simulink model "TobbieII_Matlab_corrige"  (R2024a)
settings: Solver=VariableStepAuto  StartTime=0.0  StopTime=10  RelTol=1e-3
model workspace: external: MATLAB File (data not in the file)
undefined symbols (not defined in the file or in its folder): deg, kg, m, mm, N, s, smiData, X, Y, Z
libraries: sm_lib x63, fl_lib x16, nesl_utility x9, ee_lib x2, simulink x1
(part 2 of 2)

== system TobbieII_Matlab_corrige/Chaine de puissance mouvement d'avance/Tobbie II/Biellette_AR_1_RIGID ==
  ReferenceFrame : sm_lib/Frames and Transforms/Reference Frame
  Solid : sm_lib/Body Elements/File Solid  ExtGeomFileName=Biellette AR_Défaut_sldprt.STEP  UnitType=FromFile  ExtGeomFileUnits=m  StepReaderType=HEX  ExportConvexHullGeometry=off  InertiaType=Custom  BasedOnType=DensityFromFile  Density=1000  DensityUnits=kg/m^3  Mass=smiData.Solid(2).mass  MassUnits=kg  CenterOfMass=smiData.Solid(2).CoM  CenterOfMassUnits=mm  MomentsOfInertia=smiData.Solid(2).MoI  MomentsOfInertiaUnits=kg*mm^2  ProductsOfInertia=smiData.Solid(2).PoI  ProductsOfInertiaUnits=kg*mm^2  GraphicType=FromGeometry  MarkerShape=Sphere  MarkerSize=10  GraphicVisPropType=SimpleVisualProperties  GraphicDiffuseColor=smiData.Solid(2).color  GraphicOpacity=smiData.Solid(2).opacity  GraphicSpecularColor=[0.5 0.5 0.5 1.0]  GraphicAmbientColor=[0.15 0.15 0.15 1.0]  GraphicEmissiveColor=[0.0 0.0 0.0 1.0]  GraphicShininess=75  DoExposeReferenceFrame=on  SerializedFrames=<Frames/>
  Transform : sm_lib/Frames and Transforms/Rigid Transform  RotationMethod=ArbitraryAxis  FollAlignAxisA=+X  BaseAlignAxisA=+Y  FollAlignAxisB=+Y  BaseAlignAxisB=+Z  RotationStandardAxis=+Z  RotationAngle=smiData.RigidTransform(23).angle  RotationAngleUnits=rad  RotationArbitraryAxis=smiData.RigidTransform(23).axis  RotationSequenceAxes=FollowerAxes  RotationSequence=XYX  RotationSequenceAngles=[0 0 0]  RotationSequenceAnglesUnits=deg  RotationMatrix=[1 0 0;0 1 0;0 0 1]  Quaternion=[1 0 0 0]  TranslationMethod=Cartesian  TranslationCartesianOffset=smiData.RigidTransform(23).translation  TranslationCartesianOffsetUnits=mm  TranslationStandardAxis=+Z  TranslationStandardOffset=0  TranslationStandardOffsetUnits=m  TranslationROffset=0  TranslationROffsetUnits=m  TranslationThetaOffset=0  TranslationThetaOffsetUnits=deg  TranslationZOffset=0  TranslationZOffsetUnits=m
  Transform1 : sm_lib/Frames and Transforms/Rigid Transform  RotationMethod=ArbitraryAxis  FollAlignAxisA=+X  BaseAlignAxisA=+Y  FollAlignAxisB=+Y  BaseAlignAxisB=+Z  RotationStandardAxis=+Z  RotationAngle=smiData.RigidTransform(26).angle  RotationAngleUnits=rad  RotationArbitraryAxis=smiData.RigidTransform(26).axis  RotationSequenceAxes=FollowerAxes  RotationSequence=XYX  RotationSequenceAngles=[0 0 0]  RotationSequenceAnglesUnits=deg  RotationMatrix=[1 0 0;0 1 0;0 0 1]  Quaternion=[1 0 0 0]  TranslationMethod=Cartesian  TranslationCartesianOffset=smiData.RigidTransform(26).translation  TranslationCartesianOffsetUnits=mm  TranslationStandardAxis=+Z  TranslationStandardOffset=0  TranslationStandardOffsetUnits=m  TranslationROffset=0  TranslationROffsetUnits=m  TranslationThetaOffset=0  TranslationThetaOffsetUnits=deg  TranslationZOffset=0  TranslationZOffsetUnits=m
  F1 : PMIOPort  Side=Left
  F : PMIOPort  Port=2  Side=Right
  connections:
  Solid/RConn1 -- ReferenceFrame/RConn1 -- Transform/LConn1 -- Transform1/LConn1
  Transform/RConn1 -- F/RConn1
  Transform1/RConn1 -- F1/RConn1

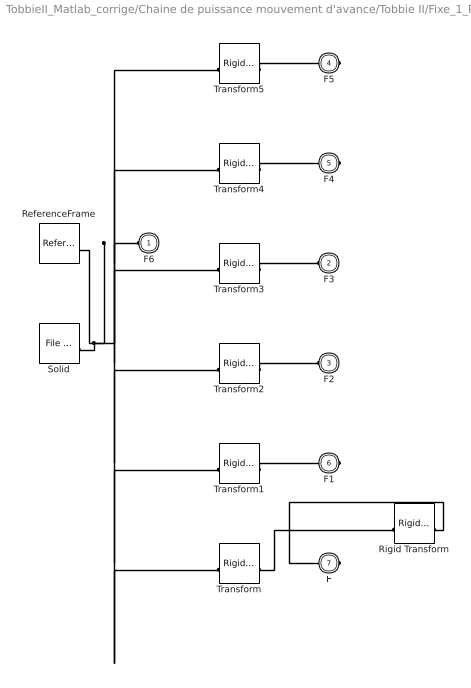
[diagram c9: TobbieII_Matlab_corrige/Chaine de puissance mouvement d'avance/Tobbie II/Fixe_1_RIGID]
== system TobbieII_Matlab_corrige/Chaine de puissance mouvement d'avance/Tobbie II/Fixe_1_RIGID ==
  ReferenceFrame : sm_lib/Frames and Transforms/Reference Frame
  Rigid Transform : sm_lib/Frames and Transforms/Rigid Transform  RotationMethod=RotationSequence  FollAlignAxisA=+X  BaseAlignAxisA=+Y  FollAlignAxisB=+Y  BaseAlignAxisB=+Z  RotationStandardAxis=+Z  RotationAngle=0  RotationAngleUnits=deg  RotationArbitraryAxis=[0 0 1]  RotationSequenceAxes=FollowerAxes  RotationSequence=XYZ  RotationSequenceAngles=[90 0 90]  RotationSequenceAnglesUnits=deg  RotationMatrix=[1 0 0;0 1 0;0 0 1]  Quaternion=[1 0 0 0]  TranslationMethod=Cartesian  TranslationCartesianOffset=[-2 0 0]  TranslationCartesianOffsetUnits=mm  TranslationStandardAxis=+Z  TranslationStandardOffset=0  TranslationStandardOffsetUnits=m  TranslationROffset=0  TranslationROffsetUnits=m  TranslationThetaOffset=0  TranslationThetaOffsetUnits=deg  TranslationZOffset=0  TranslationZOffsetUnits=m
  Solid : sm_lib/Body Elements/File Solid  ExtGeomFileName=Fixe_Défaut_sldprt.STEP  UnitType=FromFile  ExtGeomFileUnits=m  StepReaderType=HEX  ExportConvexHullGeometry=off  InertiaType=Custom  BasedOnType=DensityFromFile  Density=1000  DensityUnits=kg/m^3  Mass=smiData.Solid(5).mass  MassUnits=kg  CenterOfMass=smiData.Solid(5).CoM  CenterOfMassUnits=mm  MomentsOfInertia=smiData.Solid(5).MoI  MomentsOfInertiaUnits=kg*mm^2  ProductsOfInertia=smiData.Solid(5).PoI  ProductsOfInertiaUnits=kg*mm^2  GraphicType=FromGeometry  MarkerShape=Sphere  MarkerSize=10  GraphicVisPropType=SimpleVisualProperties  GraphicDiffuseColor=smiData.Solid(5).color  GraphicOpacity=smiData.Solid(5).opacity  GraphicSpecularColor=[0.5 0.5 0.5 1.0]  GraphicAmbientColor=[0.15 0.15 0.15 1.0]  GraphicEmissiveColor=[0.0 0.0 0.0 1.0]  GraphicShininess=75  DoExposeReferenceFrame=on  SerializedFrames=<Frames/>
  Transform : sm_lib/Frames and Transforms/Rigid Transform  RotationMethod=ArbitraryAxis  FollAlignAxisA=+X  BaseAlignAxisA=+Y  FollAlignAxisB=+Y  BaseAlignAxisB=+Z  RotationStandardAxis=+Z  RotationAngle=smiData.RigidTransform(3).angle  RotationAngleUnits=rad  RotationArbitraryAxis=smiData.RigidTransform(3).axis  RotationSequenceAxes=FollowerAxes  RotationSequence=XYX  RotationSequenceAngles=[0 0 0]  RotationSequenceAnglesUnits=deg  RotationMatrix=[1 0 0;0 1 0;0 0 1]  Quaternion=[1 0 0 0]  TranslationMethod=Cartesian  TranslationCartesianOffset=smiData.RigidTransform(3).translation  TranslationCartesianOffsetUnits=mm  TranslationStandardAxis=+Z  TranslationStandardOffset=0  TranslationStandardOffsetUnits=m  TranslationROffset=0  TranslationROffsetUnits=m  TranslationThetaOffset=0  TranslationThetaOffsetUnits=deg  TranslationZOffset=0  TranslationZOffsetUnits=m
  Transform1 : sm_lib/Frames and Transforms/Rigid Transform  RotationMethod=ArbitraryAxis  FollAlignAxisA=+X  BaseAlignAxisA=+Y  FollAlignAxisB=+Y  BaseAlignAxisB=+Z  RotationStandardAxis=+Z  RotationAngle=smiData.RigidTransform(9).angle  RotationAngleUnits=rad  RotationArbitraryAxis=smiData.RigidTransform(9).axis  RotationSequenceAxes=FollowerAxes  RotationSequence=XYX  RotationSequenceAngles=[0 0 0]  RotationSequenceAnglesUnits=deg  RotationMatrix=[1 0 0;0 1 0;0 0 1]  Quaternion=[1 0 0 0]  TranslationMethod=Cartesian  TranslationCartesianOffset=smiData.RigidTransform(9).translation  TranslationCartesianOffsetUnits=mm  TranslationStandardAxis=+Z  TranslationStandardOffset=0  TranslationStandardOffsetUnits=m  TranslationROffset=0  TranslationROffsetUnits=m  TranslationThetaOffset=0  TranslationThetaOffsetUnits=deg  TranslationZOffset=0  TranslationZOffsetUnits=m
  Transform2 : sm_lib/Frames and Transforms/Rigid Transform  RotationMethod=ArbitraryAxis  FollAlignAxisA=+X  BaseAlignAxisA=+Y  FollAlignAxisB=+Y  BaseAlignAxisB=+Z  RotationStandardAxis=+Z  RotationAngle=smiData.RigidTransform(18).angle  RotationAngleUnits=rad  RotationArbitraryAxis=smiData.RigidTransform(18).axis  RotationSequenceAxes=FollowerAxes  RotationSequence=XYX  RotationSequenceAngles=[0 0 0]  RotationSequenceAnglesUnits=deg  RotationMatrix=[1 0 0;0 1 0;0 0 1]  Quaternion=[1 0 0 0]  TranslationMethod=Cartesian  TranslationCartesianOffset=smiData.RigidTransform(18).translation  TranslationCartesianOffsetUnits=mm  TranslationStandardAxis=+Z  TranslationStandardOffset=0  TranslationStandardOffsetUnits=m  TranslationROffset=0  TranslationROffsetUnits=m  TranslationThetaOffset=0  TranslationThetaOffsetUnits=deg  TranslationZOffset=0  TranslationZOffsetUnits=m
  Transform3 : sm_lib/Frames and Transforms/Rigid Transform  RotationMethod=ArbitraryAxis  FollAlignAxisA=+X  BaseAlignAxisA=+Y  FollAlignAxisB=+Y  BaseAlignAxisB=+Z  RotationStandardAxis=+Z  RotationAngle=smiData.RigidTransform(20).angle  RotationAngleUnits=rad  RotationArbitraryAxis=smiData.RigidTransform(20).axis  RotationSequenceAxes=FollowerAxes  RotationSequence=XYX  RotationSequenceAngles=[0 0 0]  RotationSequenceAnglesUnits=deg  RotationMatrix=[1 0 0;0 1 0;0 0 1]  Quaternion=[1 0 0 0]  TranslationMethod=Cartesian  TranslationCartesianOffset=smiData.RigidTransform(20).translation  TranslationCartesianOffsetUnits=mm  TranslationStandardAxis=+Z  TranslationStandardOffset=0  TranslationStandardOffsetUnits=m  TranslationROffset=0  TranslationROffsetUnits=m  TranslationThetaOffset=0  TranslationThetaOffsetUnits=deg  TranslationZOffset=0  TranslationZOffsetUnits=m
  Transform4 : sm_lib/Frames and Transforms/Rigid Transform  RotationMethod=ArbitraryAxis  FollAlignAxisA=+X  BaseAlignAxisA=+Y  FollAlignAxisB=+Y  BaseAlignAxisB=+Z  RotationStandardAxis=+Z  RotationAngle=smiData.RigidTransform(21).angle  RotationAngleUnits=rad  RotationArbitraryAxis=smiData.RigidTransform(21).axis  RotationSequenceAxes=FollowerAxes  RotationSequence=XYX  RotationSequenceAngles=[0 0 0]  RotationSequenceAnglesUnits=deg  RotationMatrix=[1 0 0;0 1 0;0 0 1]  Quaternion=[1 0 0 0]  TranslationMethod=Cartesian  TranslationCartesianOffset=smiData.RigidTransform(21).translation  TranslationCartesianOffsetUnits=mm  TranslationStandardAxis=+Z  TranslationStandardOffset=0  TranslationStandardOffsetUnits=m  TranslationROffset=0  TranslationROffsetUnits=m  TranslationThetaOffset=0  TranslationThetaOffsetUnits=deg  TranslationZOffset=0  TranslationZOffsetUnits=m
  Transform5 : sm_lib/Frames and Transforms/Rigid Transform  RotationMethod=ArbitraryAxis  FollAlignAxisA=+X  BaseAlignAxisA=+Y  FollAlignAxisB=+Y  BaseAlignAxisB=+Z  RotationStandardAxis=+Z  RotationAngle=smiData.RigidTransform(25).angle  RotationAngleUnits=rad  RotationArbitraryAxis=smiData.RigidTransform(25).axis  RotationSequenceAxes=FollowerAxes  RotationSequence=XYX  RotationSequenceAngles=[0 0 0]  RotationSequenceAnglesUnits=deg  RotationMatrix=[1 0 0;0 1 0;0 0 1]  Quaternion=[1 0 0 0]  TranslationMethod=Cartesian  TranslationCartesianOffset=smiData.RigidTransform(25).translation  TranslationCartesianOffsetUnits=mm  TranslationStandardAxis=+Z  TranslationStandardOffset=0  TranslationStandardOffsetUnits=m  TranslationROffset=0  TranslationROffsetUnits=m  TranslationThetaOffset=0  TranslationThetaOffsetUnits=deg  TranslationZOffset=0  TranslationZOffsetUnits=m
  F6 : PMIOPort  Side=Left
  F3 : PMIOPort  Port=2  Side=Left
  F2 : PMIOPort  Port=3  Side=Left
  F5 : PMIOPort  Port=4  Side=Right
  F4 : PMIOPort  Port=5  Side=Right
  F1 : PMIOPort  Port=6  Side=Right
  F : PMIOPort  Port=7  Side=Right
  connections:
  Solid/RConn1 -- ReferenceFrame/RConn1 -- Transform/LConn1 -- Transform1/LConn1 -- Transform2/LConn1 -- Transform3/LConn1 -- Transform4/LConn1 -- Transform5/LConn1 -- F6/RConn1
  Transform/RConn1 -- Rigid Transform/LConn1
  Transform1/RConn1 -- F1/RConn1
  Transform2/RConn1 -- F2/RConn1
  Transform3/RConn1 -- F3/RConn1
  Transform4/RConn1 -- F4/RConn1
  Transform5/RConn1 -- F5/RConn1
  Rigid Transform/RConn1 -- F/RConn1

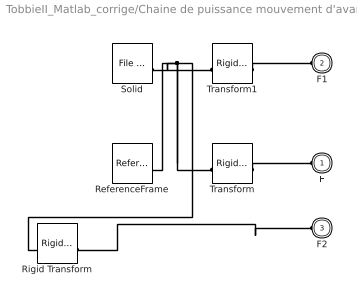
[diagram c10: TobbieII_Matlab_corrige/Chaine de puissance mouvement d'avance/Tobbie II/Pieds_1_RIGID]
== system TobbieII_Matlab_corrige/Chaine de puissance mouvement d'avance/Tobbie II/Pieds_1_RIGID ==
  ReferenceFrame : sm_lib/Frames and Transforms/Reference Frame
  Rigid Transform : sm_lib/Frames and Transforms/Rigid Transform  RotationMethod=None  FollAlignAxisA=+X  BaseAlignAxisA=+Y  FollAlignAxisB=+Y  BaseAlignAxisB=+Z  RotationStandardAxis=+Z  RotationAngle=0  RotationAngleUnits=deg  RotationArbitraryAxis=[0 0 1]  RotationSequenceAxes=FollowerAxes  RotationSequence=XYX  RotationSequenceAngles=[0 0 0]  RotationSequenceAnglesUnits=deg  RotationMatrix=[1 0 0;0 1 0;0 0 1]  Quaternion=[1 0 0 0]  TranslationMethod=Cartesian  TranslationCartesianOffset=[0 -42 0]  TranslationCartesianOffsetUnits=mm  TranslationStandardAxis=+Z  TranslationStandardOffset=0  TranslationStandardOffsetUnits=m  TranslationROffset=0  TranslationROffsetUnits=m  TranslationThetaOffset=0  TranslationThetaOffsetUnits=deg  TranslationZOffset=0  TranslationZOffsetUnits=m
  Solid : sm_lib/Body Elements/File Solid  ExtGeomFileName=Pieds_Défaut_sldprt.STEP  UnitType=FromFile  ExtGeomFileUnits=m  StepReaderType=HEX  ExportConvexHullGeometry=off  InertiaType=Custom  BasedOnType=DensityFromFile  Density=1000  DensityUnits=kg/m^3  Mass=smiData.Solid(7).mass  MassUnits=kg  CenterOfMass=smiData.Solid(7).CoM  CenterOfMassUnits=mm  MomentsOfInertia=smiData.Solid(7).MoI  MomentsOfInertiaUnits=kg*mm^2  ProductsOfInertia=smiData.Solid(7).PoI  ProductsOfInertiaUnits=kg*mm^2  GraphicType=FromGeometry  MarkerShape=Sphere  MarkerSize=10  GraphicVisPropType=SimpleVisualProperties  GraphicDiffuseColor=smiData.Solid(7).color  GraphicOpacity=smiData.Solid(7).opacity  GraphicSpecularColor=[0.5 0.5 0.5 1.0]  GraphicAmbientColor=[0.15 0.15 0.15 1.0]  GraphicEmissiveColor=[0.0 0.0 0.0 1.0]  GraphicShininess=75  DoExposeReferenceFrame=on  SerializedFrames=<Frames/>
  Transform : sm_lib/Frames and Transforms/Rigid Transform  RotationMethod=ArbitraryAxis  FollAlignAxisA=+X  BaseAlignAxisA=+Y  FollAlignAxisB=+Y  BaseAlignAxisB=+Z  RotationStandardAxis=+Z  RotationAngle=smiData.RigidTransform(2).angle  RotationAngleUnits=rad  RotationArbitraryAxis=smiData.RigidTransform(2).axis  RotationSequenceAxes=FollowerAxes  RotationSequence=XYX  RotationSequenceAngles=[0 0 0]  RotationSequenceAnglesUnits=deg  RotationMatrix=[1 0 0;0 1 0;0 0 1]  Quaternion=[1 0 0 0]  TranslationMethod=Cartesian  TranslationCartesianOffset=smiData.RigidTransform(2).translation  TranslationCartesianOffsetUnits=mm  TranslationStandardAxis=+Z  TranslationStandardOffset=0  TranslationStandardOffsetUnits=m  TranslationROffset=0  TranslationROffsetUnits=m  TranslationThetaOffset=0  TranslationThetaOffsetUnits=deg  TranslationZOffset=0  TranslationZOffsetUnits=m
  Transform1 : sm_lib/Frames and Transforms/Rigid Transform  RotationMethod=ArbitraryAxis  FollAlignAxisA=+X  BaseAlignAxisA=+Y  FollAlignAxisB=+Y  BaseAlignAxisB=+Z  RotationStandardAxis=+Z  RotationAngle=smiData.RigidTransform(8).angle  RotationAngleUnits=rad  RotationArbitraryAxis=smiData.RigidTransform(8).axis  RotationSequenceAxes=FollowerAxes  RotationSequence=XYX  RotationSequenceAngles=[0 0 0]  RotationSequenceAnglesUnits=deg  RotationMatrix=[1 0 0;0 1 0;0 0 1]  Quaternion=[1 0 0 0]  TranslationMethod=Cartesian  TranslationCartesianOffset=smiData.RigidTransform(8).translation  TranslationCartesianOffsetUnits=mm  TranslationStandardAxis=+Z  TranslationStandardOffset=0  TranslationStandardOffsetUnits=m  TranslationROffset=0  TranslationROffsetUnits=m  TranslationThetaOffset=0  TranslationThetaOffsetUnits=deg  TranslationZOffset=0  TranslationZOffsetUnits=m
  F : PMIOPort  Side=Left
  F1 : PMIOPort  Port=2  Side=Left
  F2 : PMIOPort  Port=3  Side=Left
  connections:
  Solid/RConn1 -- Rigid Transform/LConn1 -- Transform/LConn1 -- ReferenceFrame/RConn1 -- Transform1/LConn1
  Transform/RConn1 -- F/RConn1
  Transform1/RConn1 -- F1/RConn1
  Rigid Transform/RConn1 -- F2/RConn1

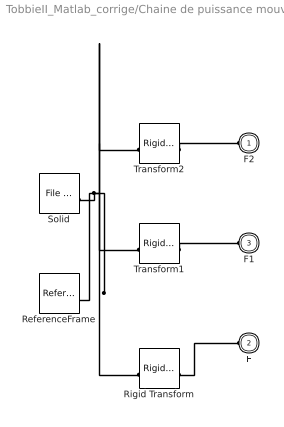
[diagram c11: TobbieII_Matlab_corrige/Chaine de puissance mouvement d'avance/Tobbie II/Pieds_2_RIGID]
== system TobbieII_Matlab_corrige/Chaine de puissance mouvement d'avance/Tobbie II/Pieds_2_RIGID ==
  ReferenceFrame : sm_lib/Frames and Transforms/Reference Frame
  Rigid Transform : sm_lib/Frames and Transforms/Rigid Transform  RotationMethod=StandardAxis  FollAlignAxisA=+X  BaseAlignAxisA=+Y  FollAlignAxisB=+Y  BaseAlignAxisB=+Z  RotationStandardAxis=+Z  RotationAngle=159.06  RotationAngleUnits=deg  RotationArbitraryAxis=[0 0 1]  RotationSequenceAxes=FollowerAxes  RotationSequence=XYX  RotationSequenceAngles=[0 0 0]  RotationSequenceAnglesUnits=deg  RotationMatrix=[1 0 0;0 1 0;0 0 1]  Quaternion=[1 0 0 0]  TranslationMethod=Cartesian  TranslationCartesianOffset=[0 -42 0]  TranslationCartesianOffsetUnits=mm  TranslationStandardAxis=+Z  TranslationStandardOffset=0  TranslationStandardOffsetUnits=m  TranslationROffset=0  TranslationROffsetUnits=m  TranslationThetaOffset=0  TranslationThetaOffsetUnits=deg  TranslationZOffset=0  TranslationZOffsetUnits=m
  Solid : sm_lib/Body Elements/File Solid  ExtGeomFileName=Pieds_Défaut_sldprt.STEP  UnitType=FromFile  ExtGeomFileUnits=m  StepReaderType=HEX  ExportConvexHullGeometry=off  InertiaType=Custom  BasedOnType=DensityFromFile  Density=1000  DensityUnits=kg/m^3  Mass=smiData.Solid(7).mass  MassUnits=kg  CenterOfMass=smiData.Solid(7).CoM  CenterOfMassUnits=mm  MomentsOfInertia=smiData.Solid(7).MoI  MomentsOfInertiaUnits=kg*mm^2  ProductsOfInertia=smiData.Solid(7).PoI  ProductsOfInertiaUnits=kg*mm^2  GraphicType=FromGeometry  MarkerShape=Sphere  MarkerSize=10  GraphicVisPropType=SimpleVisualProperties  GraphicDiffuseColor=smiData.Solid(7).color  GraphicOpacity=smiData.Solid(7).opacity  GraphicSpecularColor=[0.5 0.5 0.5 1.0]  GraphicAmbientColor=[0.15 0.15 0.15 1.0]  GraphicEmissiveColor=[0.0 0.0 0.0 1.0]  GraphicShininess=75  DoExposeReferenceFrame=on  SerializedFrames=<Frames/>
  Transform1 : sm_lib/Frames and Transforms/Rigid Transform  RotationMethod=ArbitraryAxis  FollAlignAxisA=+X  BaseAlignAxisA=+Y  FollAlignAxisB=+Y  BaseAlignAxisB=+Z  RotationStandardAxis=+Z  RotationAngle=smiData.RigidTransform(6).angle  RotationAngleUnits=rad  RotationArbitraryAxis=smiData.RigidTransform(6).axis  RotationSequenceAxes=FollowerAxes  RotationSequence=XYX  RotationSequenceAngles=[0 0 0]  RotationSequenceAnglesUnits=deg  RotationMatrix=[1 0 0;0 1 0;0 0 1]  Quaternion=[1 0 0 0]  TranslationMethod=Cartesian  TranslationCartesianOffset=smiData.RigidTransform(6).translation  TranslationCartesianOffsetUnits=mm  TranslationStandardAxis=+Z  TranslationStandardOffset=0  TranslationStandardOffsetUnits=m  TranslationROffset=0  TranslationROffsetUnits=m  TranslationThetaOffset=0  TranslationThetaOffsetUnits=deg  TranslationZOffset=0  TranslationZOffsetUnits=m
  Transform2 : sm_lib/Frames and Transforms/Rigid Transform  RotationMethod=ArbitraryAxis  FollAlignAxisA=+X  BaseAlignAxisA=+Y  FollAlignAxisB=+Y  BaseAlignAxisB=+Z  RotationStandardAxis=+Z  RotationAngle=smiData.RigidTransform(24).angle  RotationAngleUnits=rad  RotationArbitraryAxis=smiData.RigidTransform(24).axis  RotationSequenceAxes=FollowerAxes  RotationSequence=XYX  RotationSequenceAngles=[0 0 0]  RotationSequenceAnglesUnits=deg  RotationMatrix=[1 0 0;0 1 0;0 0 1]  Quaternion=[1 0 0 0]  TranslationMethod=Cartesian  TranslationCartesianOffset=smiData.RigidTransform(24).translation  TranslationCartesianOffsetUnits=mm  TranslationStandardAxis=+Z  TranslationStandardOffset=0  TranslationStandardOffsetUnits=m  TranslationROffset=0  TranslationROffsetUnits=m  TranslationThetaOffset=0  TranslationThetaOffsetUnits=deg  TranslationZOffset=0  TranslationZOffsetUnits=m
  F2 : PMIOPort  Side=Left
  F : PMIOPort  Port=2  Side=Left
  F1 : PMIOPort  Port=3  Side=Left
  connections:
  Solid/RConn1 -- ReferenceFrame/RConn1 -- Rigid Transform/LConn1 -- Transform1/LConn1 -- Transform2/LConn1
  Rigid Transform/RConn1 -- F/RConn1
  Transform1/RConn1 -- F1/RConn1
  Transform2/RConn1 -- F2/RConn1

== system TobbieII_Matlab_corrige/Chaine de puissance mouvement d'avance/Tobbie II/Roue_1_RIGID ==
  ReferenceFrame : sm_lib/Frames and Transforms/Reference Frame
  Solid : sm_lib/Body Elements/File Solid  ExtGeomFileName=Roue_Défaut_sldprt.STEP  UnitType=FromFile  ExtGeomFileUnits=m  StepReaderType=HEX  ExportConvexHullGeometry=off  InertiaType=Custom  BasedOnType=DensityFromFile  Density=1000  DensityUnits=kg/m^3  Mass=smiData.Solid(3).mass  MassUnits=kg  CenterOfMass=smiData.Solid(3).CoM  CenterOfMassUnits=mm  MomentsOfInertia=smiData.Solid(3).MoI  MomentsOfInertiaUnits=kg*mm^2  ProductsOfInertia=smiData.Solid(3).PoI  ProductsOfInertiaUnits=kg*mm^2  GraphicType=FromGeometry  MarkerShape=Sphere  MarkerSize=10  GraphicVisPropType=SimpleVisualProperties  GraphicDiffuseColor=smiData.Solid(3).color  GraphicOpacity=smiData.Solid(3).opacity  GraphicSpecularColor=[0.5 0.5 0.5 1.0]  GraphicAmbientColor=[0.15 0.15 0.15 1.0]  GraphicEmissiveColor=[0.0 0.0 0.0 1.0]  GraphicShininess=75  DoExposeReferenceFrame=on  SerializedFrames=<Frames/>
  Transform : sm_lib/Frames and Transforms/Rigid Transform  RotationMethod=ArbitraryAxis  FollAlignAxisA=+X  BaseAlignAxisA=+Y  FollAlignAxisB=+Y  BaseAlignAxisB=+Z  RotationStandardAxis=+Z  RotationAngle=smiData.RigidTransform(11).angle  RotationAngleUnits=rad  RotationArbitraryAxis=smiData.RigidTransform(11).axis  RotationSequenceAxes=FollowerAxes  RotationSequence=XYX  RotationSequenceAngles=[0 0 0]  RotationSequenceAnglesUnits=deg  RotationMatrix=[1 0 0;0 1 0;0 0 1]  Quaternion=[1 0 0 0]  TranslationMethod=Cartesian  TranslationCartesianOffset=smiData.RigidTransform(11).translation  TranslationCartesianOffsetUnits=mm  TranslationStandardAxis=+Z  TranslationStandardOffset=0  TranslationStandardOffsetUnits=m  TranslationROffset=0  TranslationROffsetUnits=m  TranslationThetaOffset=0  TranslationThetaOffsetUnits=deg  TranslationZOffset=0  TranslationZOffsetUnits=m
  Transform1 : sm_lib/Frames and Transforms/Rigid Transform  RotationMethod=ArbitraryAxis  FollAlignAxisA=+X  BaseAlignAxisA=+Y  FollAlignAxisB=+Y  BaseAlignAxisB=+Z  RotationStandardAxis=+Z  RotationAngle=smiData.RigidTransform(17).angle  RotationAngleUnits=rad  RotationArbitraryAxis=smiData.RigidTransform(17).axis  RotationSequenceAxes=FollowerAxes  RotationSequence=XYX  RotationSequenceAngles=[0 0 0]  RotationSequenceAnglesUnits=deg  RotationMatrix=[1 0 0;0 1 0;0 0 1]  Quaternion=[1 0 0 0]  TranslationMethod=Cartesian  TranslationCartesianOffset=smiData.RigidTransform(17).translation  TranslationCartesianOffsetUnits=mm  TranslationStandardAxis=+Z  TranslationStandardOffset=0  TranslationStandardOffsetUnits=m  TranslationROffset=0  TranslationROffsetUnits=m  TranslationThetaOffset=0  TranslationThetaOffsetUnits=deg  TranslationZOffset=0  TranslationZOffsetUnits=m
  F1 : PMIOPort  Side=Right
  F : PMIOPort  Port=2  Side=Right
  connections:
  Solid/RConn1 -- ReferenceFrame/RConn1 -- Transform/LConn1 -- Transform1/LConn1
  Transform/RConn1 -- F/RConn1
  Transform1/RConn1 -- F1/RConn1

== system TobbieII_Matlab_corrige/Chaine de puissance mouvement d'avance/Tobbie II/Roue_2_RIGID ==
  ReferenceFrame : sm_lib/Frames and Transforms/Reference Frame
  Solid : sm_lib/Body Elements/File Solid  ExtGeomFileName=Roue_Défaut_sldprt.STEP  UnitType=FromFile  ExtGeomFileUnits=m  StepReaderType=HEX  ExportConvexHullGeometry=off  InertiaType=Custom  BasedOnType=DensityFromFile  Density=1000  DensityUnits=kg/m^3  Mass=smiData.Solid(3).mass  MassUnits=kg  CenterOfMass=smiData.Solid(3).CoM  CenterOfMassUnits=mm  MomentsOfInertia=smiData.Solid(3).MoI  MomentsOfInertiaUnits=kg*mm^2  ProductsOfInertia=smiData.Solid(3).PoI  ProductsOfInertiaUnits=kg*mm^2  GraphicType=FromGeometry  MarkerShape=Sphere  MarkerSize=10  GraphicVisPropType=SimpleVisualProperties  GraphicDiffuseColor=smiData.Solid(3).color  GraphicOpacity=smiData.Solid(3).opacity  GraphicSpecularColor=[0.5 0.5 0.5 1.0]  GraphicAmbientColor=[0.15 0.15 0.15 1.0]  GraphicEmissiveColor=[0.0 0.0 0.0 1.0]  GraphicShininess=75  DoExposeReferenceFrame=on  SerializedFrames=<Frames/>
  Transform : sm_lib/Frames and Transforms/Rigid Transform  RotationMethod=ArbitraryAxis  FollAlignAxisA=+X  BaseAlignAxisA=+Y  FollAlignAxisB=+Y  BaseAlignAxisB=+Z  RotationStandardAxis=+Z  RotationAngle=smiData.RigidTransform(13).angle  RotationAngleUnits=rad  RotationArbitraryAxis=smiData.RigidTransform(13).axis  RotationSequenceAxes=FollowerAxes  RotationSequence=XYX  RotationSequenceAngles=[0 0 0]  RotationSequenceAnglesUnits=deg  RotationMatrix=[1 0 0;0 1 0;0 0 1]  Quaternion=[1 0 0 0]  TranslationMethod=Cartesian  TranslationCartesianOffset=smiData.RigidTransform(13).translation  TranslationCartesianOffsetUnits=mm  TranslationStandardAxis=+Z  TranslationStandardOffset=0  TranslationStandardOffsetUnits=m  TranslationROffset=0  TranslationROffsetUnits=m  TranslationThetaOffset=0  TranslationThetaOffsetUnits=deg  TranslationZOffset=0  TranslationZOffsetUnits=m
  Transform1 : sm_lib/Frames and Transforms/Rigid Transform  RotationMethod=ArbitraryAxis  FollAlignAxisA=+X  BaseAlignAxisA=+Y  FollAlignAxisB=+Y  BaseAlignAxisB=+Z  RotationStandardAxis=+Z  RotationAngle=smiData.RigidTransform(19).angle  RotationAngleUnits=rad  RotationArbitraryAxis=smiData.RigidTransform(19).axis  RotationSequenceAxes=FollowerAxes  RotationSequence=XYX  RotationSequenceAngles=[0 0 0]  RotationSequenceAnglesUnits=deg  RotationMatrix=[1 0 0;0 1 0;0 0 1]  Quaternion=[1 0 0 0]  TranslationMethod=Cartesian  TranslationCartesianOffset=smiData.RigidTransform(19).translation  TranslationCartesianOffsetUnits=mm  TranslationStandardAxis=+Z  TranslationStandardOffset=0  TranslationStandardOffsetUnits=m  TranslationROffset=0  TranslationROffsetUnits=m  TranslationThetaOffset=0  TranslationThetaOffsetUnits=deg  TranslationZOffset=0  TranslationZOffsetUnits=m
  F1 : PMIOPort  Side=Right
  F : PMIOPort  Port=2  Side=Right
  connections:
  Solid/RConn1 -- ReferenceFrame/RConn1 -- Transform/LConn1 -- Transform1/LConn1
  Transform/RConn1 -- F/RConn1
  Transform1/RConn1 -- F1/RConn1

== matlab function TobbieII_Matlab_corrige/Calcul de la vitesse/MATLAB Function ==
function v = CalculVitesse(G1xMax, G1xMin, G2xMax, G2xMin, t)

    % Distance parcourue
    d = abs(G1xMax - G1xMin) + abs(G2xMax - G2xMin);

    % Vitesse
    v = d / t;
end
